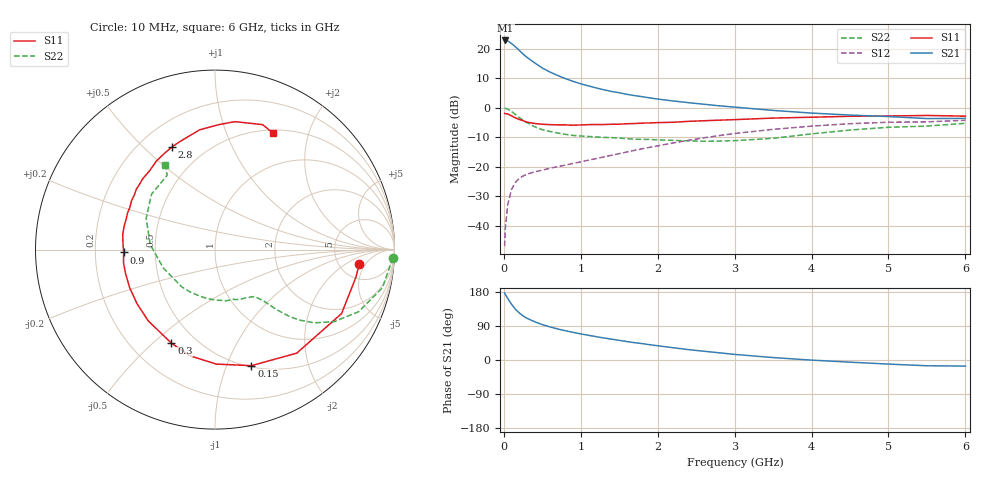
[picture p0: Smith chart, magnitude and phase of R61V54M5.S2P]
! SIEMENS Small Signal Semiconductors
! BFR193
! Si NPN RF Bipolar Junction Transistor in SOT23
! VCE = 1.5 V  IC = 4.5 mA
! Common Emitter S-Parameters:  May  1996
# GHz  S  MA  R  50
!  f  S11  S21  S12  S22
! GHz  MAG  ANG  MAG  ANG  MAG  ANG  MAG  ANG
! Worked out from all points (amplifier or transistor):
!   36 points, 10 MHz to 6 GHz, reference 50 ohm
!   highest |S21| = 22.9 dB at 20 MHz (marker M1)
!   |S21| within 3 dB of that: start of sweep to 185.7 MHz
!   unconditionally stable (mu >= 1): 895.9 MHz to 2.081 GHz
!   at 250 MHz: K = 0.40, MSG = 20.7 dB, |S12| = -23.1 dB
!   at 1.4 GHz: K = 1.08, MAG = 9.1 dB, |S12| = -16.1 dB
!   at 6 GHz: K = 0.98, MSG = 0.3 dB, |S12| = -4.2 dB
!   S11 on the Smith chart (normalised r, x): 10 MHz: 7.77, -3.52; 150 MHz: 0.51, -1.23; 300 MHz: 0.37, -0.57; 900 MHz: 0.33, -0.01; 2.8 GHz: 0.33, +0.62; 6 GHz: 0.54, +1.47
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0.01  0.8075 -5.6  13.94 176.7  0.0045 86.4  0.9913 -2.6
0.02  0.8002 -11.0  13.99 172.8  0.0092 83.6  0.9805 -5.1
0.05  0.7902 -26.8  13.77 162.5  0.0228 76.7  0.9569 -12.8
0.1  0.7351 -51.7  12.39 147.3  0.0414 65.3  0.8717 -23.4
0.15  0.6778 -72.6  10.93 133.9  0.0544 57.1  0.7755 -31.2
0.2  0.6378 -89.4  9.519 124.3  0.0636 51.7  0.6876 -36.4
0.25  0.6076 -103.4  8.219 116.5  0.07 47.8  0.6175 -39.6
0.3  0.5749 -115.0  7.256 110.2  0.0751 46.0  0.5625 -41.8
0.4  0.5443 -133.1  5.829 101.0  0.0822 44.2  0.479 -44.3
0.5  0.5286 -145.4  4.762 93.5  0.0879 44.5  0.4278 -45.5
0.6  0.5206 -156.0  4.065 87.3  0.0947 45.0  0.3982 -46.4
0.7  0.516 -164.9  3.56 81.9  0.1005 46.5  0.3751 -47.6
0.9  0.5093 -178.2  2.829 73.0  0.1142 50.0  0.3412 -50.2
1.1  0.5208 170.7  2.366 65.2  0.1298 52.8  0.3278 -54.2
1.3  0.5229 161.6  2.034 58.2  0.1476 54.8  0.316 -58.7
1.6  0.5394 149.4  1.701 48.6  0.1788 56.5  0.3014 -67.5
2.2  0.5711 129.5  1.314 32.4  0.2546 55.0  0.2811 -89.7
2.8  0.6203 112.6  1.087 19.0  0.3392 48.7  0.2737 -120.2
3.5  0.6728 97.3  0.908 6.4  0.4328 37.5  0.3055 -160.3
4.5  0.7214 81.2  0.757 -5.7  0.54 20.7  0.4218 155.4
5.5  0.7451 69.1  0.66 -15.2  0.5809 3.8  0.4921 122.8
6  0.7253 63.6  0.664 -16.1  0.6169 -1.1  0.5477 120.3
